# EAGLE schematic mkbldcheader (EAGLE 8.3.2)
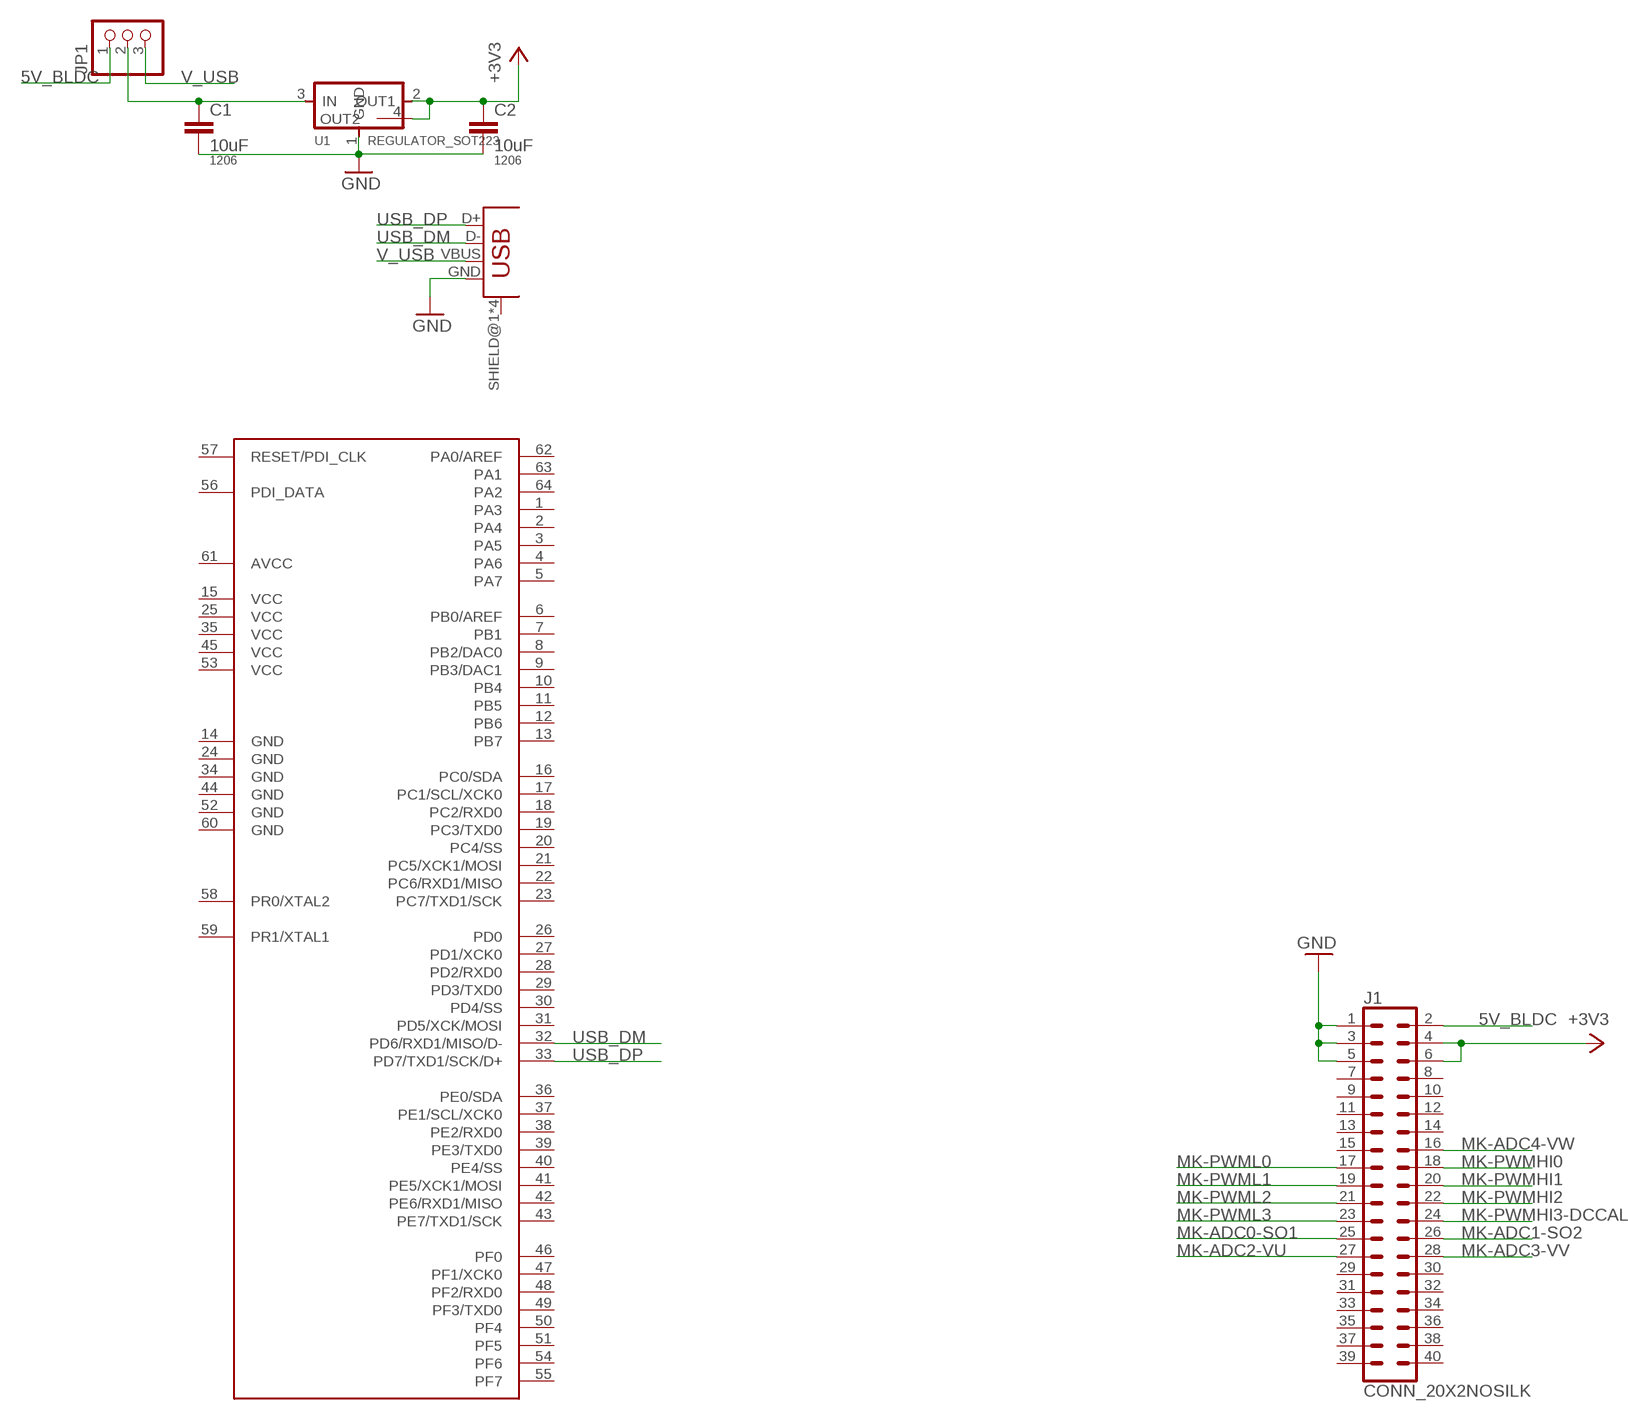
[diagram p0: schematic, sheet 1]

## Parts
C1  10uF  CAP1206  [1206]
C2  10uF  CAP1206  [1206]
J1  CONN_20X2NOSILK  [2X20_NOSILK]
JP1  PINHD-1X3  [1X03]
U1  REGULATOR_SOT223  [SOT223]
U$1  ATXMEGA_A3U  [TQFP64_14X14MM-013THIN]
U$2  USB_MINIB  [USB_MINIB]

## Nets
5V_BLDC: J1.2 JP1.1
+3V3: C2.1 J1.4 J1.6 U1.2(OUT1) U1.4(OUT2)
GND: C1.2 C2.2 J1.1 J1.3 J1.5 U1.1(GND) U$2.GND
MK-ADC0-SO1: J1.25
MK-ADC1-SO2: J1.26
MK-ADC2-VU: J1.27
MK-ADC3-VV: J1.28
MK-ADC4-VW: J1.16
MK-PWMHI0: J1.18
MK-PWMHI1: J1.20
MK-PWMHI2: J1.22
MK-PWMHI3-DCCAL: J1.24
MK-PWML0: J1.17
MK-PWML1: J1.19
MK-PWML2: J1.21
MK-PWML3: J1.23
N$4: C1.1 JP1.2 U1.3(IN)
USB_DM: U$1.32(PD6/RXD1/MISO/D-) U$2.D-
USB_DP: U$1.33(PD7/TXD1/SCK/D+) U$2.D+
V_USB: JP1.3 U$2.VBUS
Unconnected: J1.7 J1.8 J1.9 J1.10 J1.11 J1.12 J1.13 J1.14 J1.15 J1.29 J1.30 J1.31 J1.32 J1.33 J1.34 J1.35 J1.36 J1.37 J1.38 J1.39 J1.40 U$1.1(PA3) U$1.2(PA4) U$1.3(PA5) U$1.4(PA6) U$1.5(PA7) U$1.6(PB0/AREF) U$1.7(PB1) U$1.8(PB2/DAC0) U$1.9(PB3/DAC1) U$1.10(PB4) U$1.11(PB5) U$1.12(PB6) U$1.13(PB7) U$1.14(GND) U$1.15(VCC) U$1.16(PC0/SDA) U$1.17(PC1/SCL/XCK0) U$1.18(PC2/RXD0) U$1.19(PC3/TXD0) U$1.20(PC4/SS) U$1.21(PC5/XCK1/MOSI) U$1.22(PC6/RXD1/MISO) U$1.23(PC7/TXD1/SCK) U$1.24(GND) U$1.25(VCC) U$1.26(PD0) U$1.27(PD1/XCK0) U$1.28(PD2/RXD0) U$1.29(PD3/TXD0) U$1.30(PD4/SS) U$1.31(PD5/XCK/MOSI) U$1.34(GND) U$1.35(VCC) U$1.36(PE0/SDA) U$1.37(PE1/SCL/XCK0) U$1.38(PE2/RXD0) U$1.39(PE3/TXD0) U$1.40(PE4/SS) U$1.41(PE5/XCK1/MOSI) U$1.42(PE6/RXD1/MISO) U$1.43(PE7/TXD1/SCK) U$1.44(GND) U$1.45(VCC) U$1.46(PF0) U$1.47(PF1/XCK0) U$1.48(PF2/RXD0) U$1.49(PF3/TXD0) U$1.50(PF4) U$1.51(PF5) U$1.52(GND) U$1.53(VCC) U$1.54(PF6) U$1.55(PF7) U$1.56(PDI_DATA) U$1.57(RESET/PDI_CLK) U$1.58(PR0/XTAL2) U$1.59(PR1/XTAL1) U$1.60(GND) U$1.61(AVCC) U$1.62(PA0/AREF) U$1.63(PA1) U$1.64(PA2) U$2.SHIELD@1(SHIELD) U$2.SHIELD@2(SHIELD) U$2.SHIELD@3(SHIELD) U$2.SHIELD@4(SHIELD)

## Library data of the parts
C1 C2 = borkedlabs-passives:CAP: Capacitor; PACKAGE: 1206
J1 = SparkFun-Connectors:CONN_20X2: Multi connection point. Often used as Generic Header-pin footprint for 0.1 inch spaced/style header connections On any of the 0.1 inch spaced packages, you can populate with these: Break Away Headers - Straight (PRT-00116) Break Away Male Headers - Right Angle (PRT-00553) Female Headers (PRT-00115)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
JP1 = pinhead:PINHD-1X3: PIN HEADER
U1 = fab:REGULATOR_SOT223
U$1 = fab:ATXMEGA_A3U
U$2 = fab:USB_MINIB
